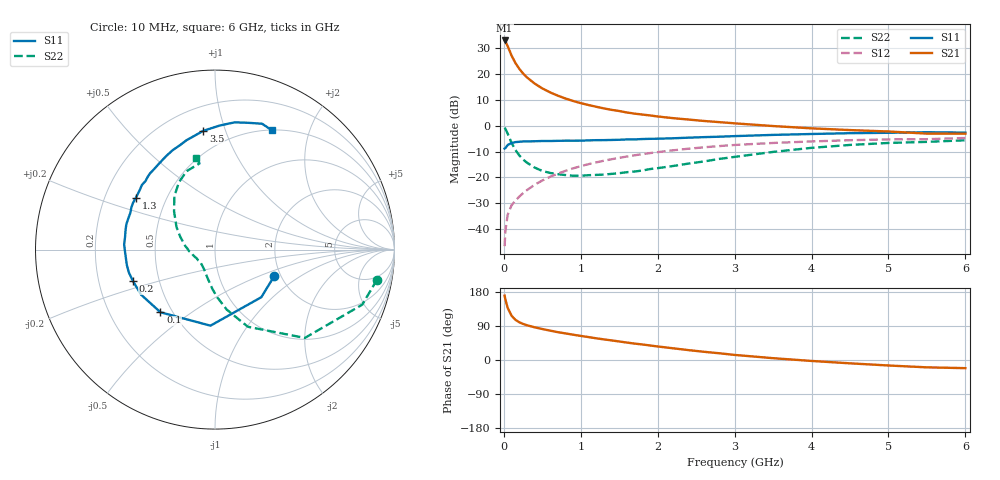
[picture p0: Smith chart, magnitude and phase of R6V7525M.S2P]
! SIEMENS Small Signal Semiconductors
! BFR193
! Si NPN RF Bipolar Junction Transistor in SOT23
! VCE = 0.75 V  IC = 25 mA
! Common Emitter S-Parameters:  May  1996
# GHz  S  MA  R  50
!  f  S11  S21  S12  S22
! GHz  MAG  ANG  MAG  ANG  MAG  ANG  MAG  ANG
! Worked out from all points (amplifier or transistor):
!   36 points, 10 MHz to 6 GHz, reference 50 ohm
!   highest |S21| = 33.0 dB at 10 MHz (marker M1)
!   |S21| within 3 dB of that: start of sweep to 60.82 MHz
!   unconditionally stable (mu >= 1): 418 MHz to 2.293 GHz
!   at 250 MHz: K = 0.90, MSG = 23.1 dB, |S12| = -26.1 dB
!   at 1.4 GHz: K = 1.04, MAG = 8.3 dB, |S12| = -12.9 dB
!   at 6 GHz: K = 0.99, MSG = 0.8 dB, |S12| = -4.7 dB
!   S11 on the Smith chart (normalised r, x): 10 MHz: 1.84, -0.63; 100 MHz: 0.43, -0.38; 200 MHz: 0.35, -0.16; 1.3 GHz: 0.33, +0.27; 3.5 GHz: 0.35, +0.84; 6 GHz: 0.50, +1.46
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0.01  0.3615 -24.2  44.47 169.8  0.0047 82.7  0.9182 -10.5
0.02  0.37 -45.8  42.91 160.0  0.0092 76.2  0.876 -20.5
0.05  0.4246 -93.4  34.43 137.4  0.019 64.1  0.702 -44.5
0.1  0.4629 -131.0  22.77 116.9  0.029 59.2  0.4675 -66.9
0.15  0.4824 -148.6  16.34 106.1  0.0356 59.4  0.341 -78.9
0.2  0.4895 -158.8  12.65 99.6  0.0425 62.2  0.2682 -87.0
0.25  0.4969 -165.3  10.23 95.2  0.0497 63.9  0.2222 -93.4
0.3  0.4986 -170.2  8.604 91.7  0.0569 65.7  0.1935 -98.0
0.4  0.5009 -178.0  6.538 86.3  0.0721 67.1  0.1558 -107.0
0.5  0.5069 176.8  5.262 81.7  0.0874 67.7  0.1334 -114.8
0.6  0.5062 171.7  4.42 77.6  0.1027 67.8  0.1224 -121.0
0.7  0.5105 167.3  3.821 73.5  0.1185 67.1  0.1159 -126.5
0.9  0.5133 160.0  3.007 66.8  0.1499 65.3  0.108 -138.3
1.1  0.5214 153.5  2.514 60.5  0.1807 63.0  0.1107 -146.8
1.3  0.5269 146.9  2.163 54.4  0.2105 60.0  0.1136 -155.4
1.7  0.5439 135.4  1.713 43.3  0.2681 54.1  0.1303 -170.9
2.2  0.5722 122.8  1.4 30.9  0.3351 45.9  0.1666 173.2
3  0.6297 104.6  1.112 13.4  0.4245 32.5  0.25 149.3
3.5  0.665 95.6  0.986 4.8  0.4646 24.3  0.3118 137.0
4.5  0.7175 81.2  0.824 -8.8  0.5249 10.3  0.4255 118.2
5.5  0.7487 69.5  0.704 -19.4  0.5492 -2.8  0.4875 100.2
6  0.7366 64.5  0.702 -21.5  0.5799 -6.7  0.5233 101.4
